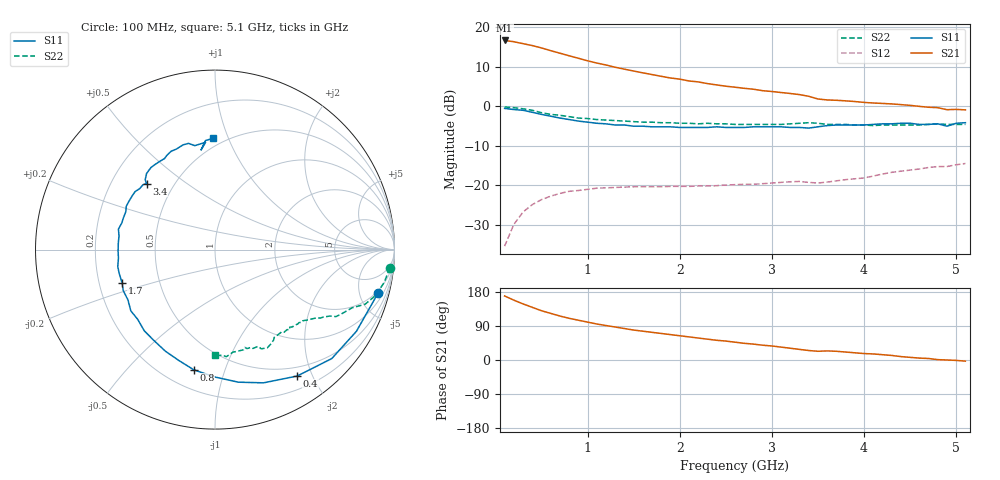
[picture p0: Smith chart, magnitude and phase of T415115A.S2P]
!AT-41511
!S-PARAMETERS at Vce=5V  Ic=2mA.  LAST UPDATED 01-25-95
# ghz s ma r 50
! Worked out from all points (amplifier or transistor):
!   51 points, 100 MHz to 5.1 GHz, reference 50 ohm
!   highest |S21| = 16.7 dB at 100 MHz (marker M1)
!   |S21| within 3 dB of that: start of sweep to 665.2 MHz
!   unconditionally stable (mu >= 1): 2.211 GHz to 5.06 GHz
!   at 900 MHz: K = 0.48, MSG = 16.7 dB, |S12| = -21.3 dB
!   at 2.6 GHz: K = 1.11, MAG = 10.3 dB, |S12| = -19.8 dB
!   at 5.1 GHz: K = 0.98, MSG = 6.8 dB, |S12| = -14.5 dB
!   lowest NFmin = 0.80 dB at 100 MHz
!   S11 on the Smith chart (normalised r, x): 100 MHz: 1.72, -7.19; 400 MHz: 0.37, -1.78; 800 MHz: 0.32, -0.79; 1.7 GHz: 0.30, -0.16; 3.4 GHz: 0.35, +0.36; 5.1 GHz: 0.44, +0.88
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0.1  0.94 -15.0  6.807 169.0  0.017 82.0  0.98 -6.0
0.2  0.91 -30.0  6.558 158.0  0.032 73.0  0.96 -11.0
0.3  0.89 -43.0  6.2 148.0  0.046 65.0  0.93 -16.0
0.4  0.84 -57.0  5.865 139.0  0.057 59.0  0.89 -20.0
0.5  0.79 -70.0  5.475 130.0  0.066 53.0  0.83 -23.0
0.7  0.71 -90.0  4.696 116.0  0.079 44.0  0.77 -29.0
0.8  0.68 -100.0  4.357 110.0  0.084 41.0  0.74 -30.0
1  0.63 -116.0  3.764 100.0  0.089 36.0  0.7 -33.0
1.1  0.61 -124.0  3.525 95.0  0.092 34.0  0.68 -34.0
1.3  0.58 -138.0  3.119 87.0  0.094 31.0  0.66 -36.0
1.5  0.56 -150.0  2.795 79.0  0.096 29.0  0.64 -38.0
1.7  0.55 -160.0  2.521 73.0  0.096 29.0  0.63 -40.0
1.8  0.55 -166.0  2.394 70.0  0.096 29.0  0.62 -41.0
2.2  0.54 176.0  2.037 58.0  0.098 29.0  0.6 -46.0
2.6  0.54 161.0  1.744 47.0  0.102 32.0  0.59 -51.0
3.4  0.53 136.0  1.338 25.0  0.109 34.0  0.62 -62.0
3.5  0.55 135.0  1.237 23.0  0.107 37.0  0.61 -65.0
3.7  0.58 128.0  1.191 23.0  0.114 42.0  0.59 -67.0
4.3  0.6 111.0  1.072 12.0  0.146 47.0  0.58 -75.0
4.8  0.6 95.0  0.961 1.0  0.173 45.0  0.6 -84.0
4.9  0.56 98.0  0.906 0.0  0.173 44.0  0.59 -86.0
5.1  0.62 91.0  0.901 -3.0  0.189 44.0  0.59 -90.0
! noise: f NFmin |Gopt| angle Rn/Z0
0.1  0.8  0.56  6  0.27
0.9  1.2  0.43  60  0.23
1.8  1.8  0.38  120  0.17
2.4  2.2  0.38  155  0.12
